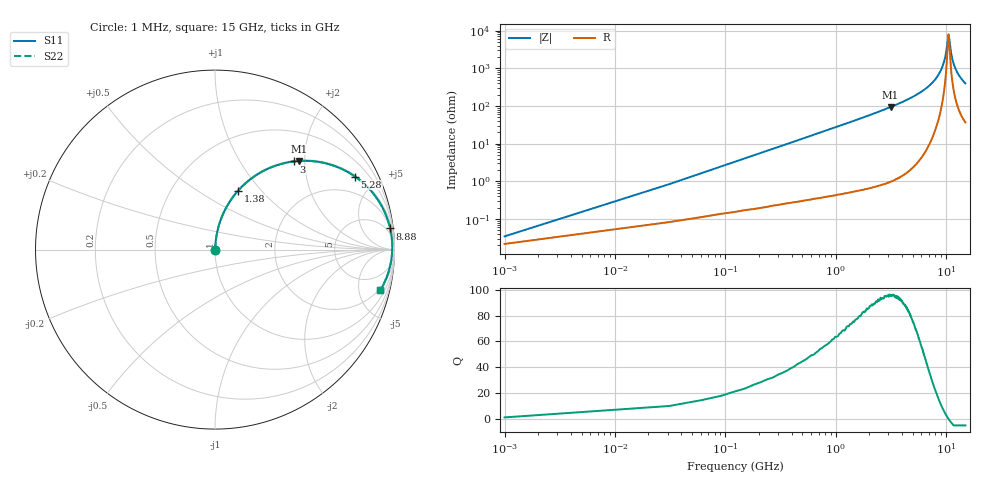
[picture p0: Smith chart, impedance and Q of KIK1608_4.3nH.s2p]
!version-2
!date-01.2022
!Series
# MHz S RI R 50
!Freq ReS11 ImS11 ReS21 ImS21 ReS12 ImS12 ReS22 ImS22
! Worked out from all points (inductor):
!   501 points, 1 MHz to 15 GHz, reference 50 ohm
!   read as one part in series: L = 4.3 nH near 61 MHz
!   highest Q = 96 at 3.15 GHz (marker M1), where L = 4.72 nH
!   self-resonance near 10.53 GHz
!   S11 on the Smith chart (normalised r, x): 1 MHz: 1.00, +0.00; 1.38 GHz: 1.01, +0.76; 3 GHz: 1.02, +1.76; 5.28 GHz: 1.05, +3.81; 8.88 GHz: 2, +16; 15 GHz: 1.73, -7.91
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1  0.000239 0.00027  0.9998 -0.00027  0.9998 -0.00027  0.000239 0.00027
91  0.00195 0.0245  0.998 -0.0245  0.998 -0.0245  0.00195 0.0245
151  0.00336 0.0406  0.9966 -0.0406  0.9966 -0.0406  0.00336 0.0406
271  0.00756 0.0726  0.9924 -0.0726  0.9924 -0.0726  0.00756 0.0726
451  0.0174 0.1196  0.9826 -0.1196  0.9826 -0.1196  0.0174 0.1196
691  0.0372 0.1799  0.9628 -0.1799  0.9628 -0.1799  0.0372 0.1799
1380  0.1293 0.3288  0.8707 -0.3288  0.8707 -0.3288  0.1293 0.3288
2520  0.3445 0.4698  0.6555 -0.4698  0.6555 -0.4698  0.3445 0.4698
3000  0.4383 0.491  0.5617 -0.491  0.5617 -0.491  0.4383 0.491
3150  0.4666 0.4937  0.5334 -0.4937  0.5334 -0.4937  0.4666 0.4937
5010  0.7505 0.4261  0.2495 -0.4261  0.2495 -0.4261  0.7505 0.4261
5280  0.7804 0.4069  0.2196 -0.4069  0.2196 -0.4069  0.7804 0.4069
7530  0.938 0.2244  0.062 -0.2244  0.062 -0.2244  0.938 0.2244
8880  0.9759 0.1177  0.0241 -0.1177  0.0241 -0.1177  0.9759 0.1177
9540  0.9843 0.0692  0.0157 -0.0692  0.0157 -0.0692  0.9843 0.0692
10020  0.9871 0.0357  0.0129 -0.0357  0.0129 -0.0357  0.9871 0.0357
10440  0.9876 0.00759  0.0124 -0.00759  0.0124 -0.00759  0.9876 0.00759
10560  0.9874 -0.000213  0.0126 0.000213  0.0126 0.000213  0.9874 -0.000213
11010  0.9858 -0.0286  0.0142 0.0286  0.0142 0.0286  0.9858 -0.0286
11340  0.9836 -0.0486  0.0164 0.0486  0.0164 0.0486  0.9836 -0.0486
12510  0.9701 -0.1139  0.0299 0.1139  0.0299 0.1139  0.9701 -0.1139
15000  0.9219 -0.226  0.0781 0.226  0.0781 0.226  0.9219 -0.226
